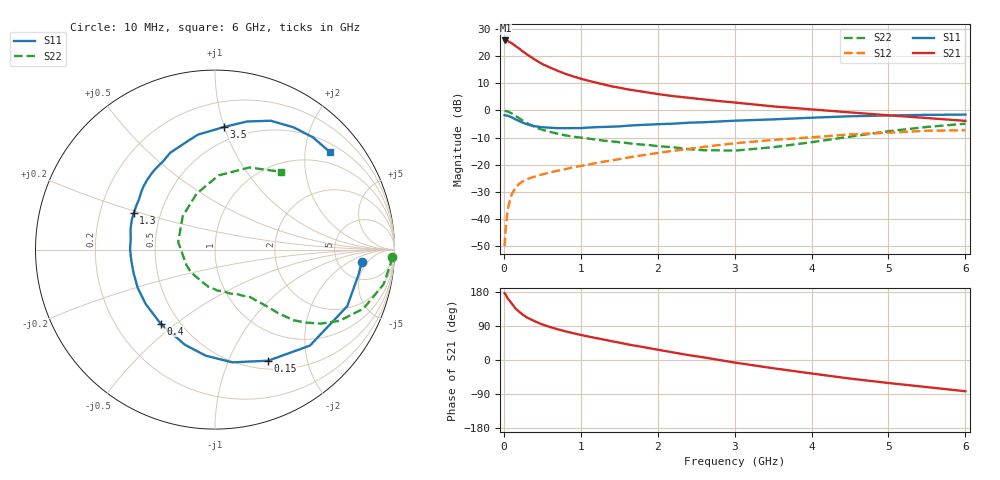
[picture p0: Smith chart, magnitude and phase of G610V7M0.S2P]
! SIEMENS Small Signal Semiconductors
! BFG193
! Si NPN RF Bipolar Junction Transistor in SOT223
! VCE = 10 V  IC = 7 mA
! Common Emitter S-Parameters:  August  1996
# GHz  S  MA  R  50
!  f  S11  S21  S12  S22
! GHz  MAG  ANG  MAG  ANG  MAG  ANG  MAG  ANG
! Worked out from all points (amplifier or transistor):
!   36 points, 10 MHz to 6 GHz, reference 50 ohm
!   highest |S21| = 25.9 dB at 20 MHz (marker M1)
!   |S21| within 3 dB of that: start of sweep to 198.9 MHz
!   unconditionally stable (mu >= 1): 1.036 GHz to 2.561 GHz
!   at 250 MHz: K = 0.41, MSG = 23.9 dB, |S12| = -26.1 dB
!   at 1.4 GHz: K = 1.08, MAG = 12.0 dB, |S12| = -18.5 dB
!   at 6 GHz: K = 0.85, MSG = 1.7 dB, |S12| = -7.3 dB
!   S11 on the Smith chart (normalised r, x): 10 MHz: 8.52, -3.64; 150 MHz: 0.60, -1.41; 400 MHz: 0.40, -0.44; 1.3 GHz: 0.35, +0.19; 3.5 GHz: 0.39, +1.00; 6 GHz: 0.69, +2.56
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0.01  0.8197 -4.9  19.71 176.1  0.0031 90.9  0.9858 -2.4
0.02  0.8124 -9.7  19.73 173.8  0.0058 81.4  0.9813 -4.8
0.05  0.8014 -23.2  19.22 162.8  0.0149 76.7  0.9586 -11.7
0.1  0.7522 -45.3  17.65 149.8  0.0277 69.0  0.8901 -21.7
0.15  0.6864 -64.4  15.67 136.4  0.0372 59.4  0.7986 -29.8
0.2  0.6354 -81.3  13.93 127.2  0.0441 54.9  0.7192 -35.0
0.25  0.5929 -95.1  12.26 118.9  0.0496 50.5  0.6435 -39.1
0.3  0.5562 -107.5  10.91 112.3  0.0536 48.5  0.5876 -42.0
0.4  0.5119 -126.3  8.789 102.4  0.0601 45.6  0.4978 -45.2
0.5  0.491 -141.9  7.244 93.8  0.0658 44.3  0.4395 -47.1
0.6  0.4805 -153.6  6.224 87.1  0.0716 44.0  0.4022 -48.8
0.7  0.472 -164.1  5.419 81.1  0.0768 44.3  0.3723 -50.7
0.9  0.4733 179.6  4.274 70.8  0.0891 44.5  0.3285 -53.5
1.1  0.4837 166.7  3.546 61.9  0.1 44.5  0.3018 -58.7
1.3  0.4967 156.0  3.029 53.8  0.1134 43.9  0.2769 -63.5
1.6  0.5228 141.6  2.474 41.6  0.1341 41.5  0.2506 -73.9
2.2  0.5702 120.6  1.844 20.0  0.1798 34.3  0.2095 -100.6
2.8  0.6272 103.1  1.494 0.0  0.2302 24.3  0.1834 -138.1
3.5  0.6852 85.7  1.191 -21.7  0.2849 9.3  0.2095 168.4
4.5  0.7824 66.6  0.922 -49.0  0.3605 -10.5  0.3281 108.2
5.5  0.8302 48.8  0.726 -71.5  0.4221 -35.6  0.4964 67.2
6  0.8398 40.3  0.643 -82.5  0.4318 -50.2  0.5695 49.5
